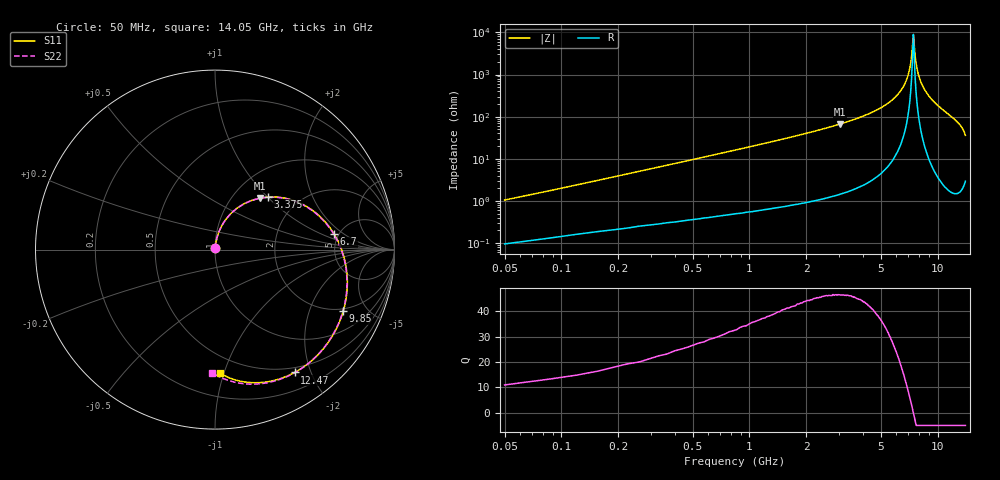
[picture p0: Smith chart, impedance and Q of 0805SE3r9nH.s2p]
! AVX Thin Film Operation		Date: May 2002
! Description: Accu-L® Series, Thin Film, SMD, RF Inductors
! Part Number: L08053R9CEWTR
! 50 MHz  -  14.05 GHz
! Serial Measurements
# mhz S db R 50
!	S11		S21		S12		S22
!	dB	Phase	dB	Phase	dB	Phase	dB	Phase
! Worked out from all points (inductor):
!   401 points, 50 MHz to 14.05 GHz, reference 50 ohm
!   read as 1/Y11, port 2 shorted: L = 3.12 nH near 120 MHz
!   highest Q = 46.4 at 3.025 GHz (marker M1), where L = 3.5 nH
!   self-resonance near 7.435 GHz
!   S11 on the Smith chart (normalised r, x): 50 MHz: 1.00, +0.02; 3.375 GHz: 1.42, +1.00; 6.7 GHz: 4.59, +1.43; 9.85 GHz: 1.87, -3.44; 12.47 GHz: 0.43, -1.76; 14.05 GHz: 0.37, -0.97
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50  -41.93 83.0  -0.01 -0.7  -0.01 -0.7  -41.93 83.0
190  -31.17 83.0  -0.02 -2.7  -0.02 -2.7  -31.17 83.0
295  -27.50 82.3  -0.03 -4.1  -0.03 -4.1  -27.50 82.3
470  -23.60 80.6  -0.05 -6.5  -0.05 -6.5  -23.60 80.5
680  -20.50 78.2  -0.08 -9.3  -0.08 -9.3  -20.50 78.1
995  -17.32 74.4  -0.13 -13.5  -0.13 -13.5  -17.32 74.3
1380  -14.61 69.5  -0.21 -18.6  -0.21 -18.6  -14.61 69.5
1835  -12.29 63.8  -0.33 -24.5  -0.33 -24.5  -12.29 63.7
2395  -10.19 56.8  -0.51 -31.7  -0.51 -31.7  -10.19 56.7
3025  -8.43 49.1  -0.76 -39.6  -0.76 -39.6  -8.43 48.9
3375  -7.64 44.8  -0.92 -43.9  -0.92 -43.9  -7.64 44.6
4740  -5.38 28.9  -1.60 -60.1  -1.60 -60.1  -5.38 28.6
6700  -3.48 7.4  -2.74 -81.8  -2.74 -81.8  -3.48 6.9
7050  -3.24 3.7  -2.95 -85.6  -2.95 -85.6  -3.24 3.2
8240  -2.60 -8.8  -3.65 -98.1  -3.65 -98.1  -2.60 -9.4
9395  -2.15 -20.8  -4.30 -110.3  -4.30 -110.3  -2.15 -21.6
9850  -2.02 -25.7  -4.53 -115.2  -4.53 -115.2  -2.02 -26.4
10830  -1.81 -36.4  -4.96 -126.1  -4.96 -126.1  -1.81 -37.4
11740  -1.72 -47.2  -5.19 -137.2  -5.19 -137.2  -1.72 -48.4
12475  -1.77 -57.0  -5.17 -147.5  -5.17 -147.5  -1.77 -58.6
13420  -2.20 -72.9  -4.56 -164.7  -4.56 -164.7  -2.21 -75.3
14050  -3.25 -87.8  -3.50 177.9  -3.50 177.9  -3.28 -91.4
